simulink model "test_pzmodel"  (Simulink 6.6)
settings: Solver=ode45  StartTime=0.0  StopTime=10.0  RelTol=1e-3
libraries: sltpda x11

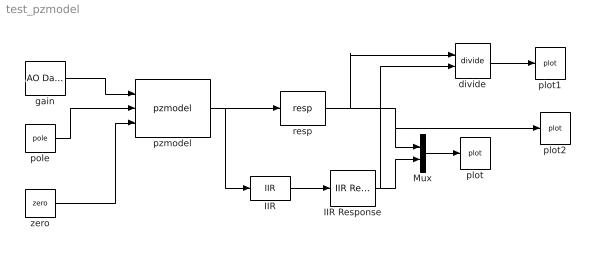
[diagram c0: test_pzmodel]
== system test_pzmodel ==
  IIR : sltpda/Pole//zero Modelling/IIR  SystemSampleTime=-1  fs=10000
  IIR Response : sltpda/Signal Processing blocks/Digital filtering/IIR Response  SystemSampleTime=-1  f1=0.1  f2=10000  nf=10000
  Mux : Mux  Inputs=2
  divide : sltpda/math blocks/divide  Tag=mrdivide  SystemSampleTime=-1
  gain : sltpda/AO class/AO Data  Tag=ao  SystemSampleTime=-1  vals=5
  plot : sltpda/AO class/plot  Tag=plot  Description=Plot an analysis object.  SystemSampleTime=-1  xscale=linear  yscale=linear
  plot1 : sltpda/AO class/plot  Tag=plot  Description=Plot an analysis object.  SystemSampleTime=-1  xscale=linear  yscale=linear
  plot2 : sltpda/AO class/plot  Tag=plot  Description=Plot an analysis object.  SystemSampleTime=-1  xscale=linear  yscale=linear
  pole : sltpda/Pole//zero Modelling/pole  Tag=pole  SystemSampleTime=-1  polef=1  poleQ=10
  pzmodel : sltpda/Pole//zero Modelling/pzmodel  SystemSampleTime=-1
  resp : sltpda/Pole//zero Modelling/resp  SystemSampleTime=-1  scale=linear
  zero : sltpda/Pole//zero Modelling/zero  Tag=zero  SystemSampleTime=-1  zerof=40  zeroQ=15
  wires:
  pole/1 -> pzmodel/2
  zero/1 -> pzmodel/3
  gain/1 -> pzmodel/1
  pzmodel/1 -> resp/1, IIR/1
  resp/1 -> divide/1, Mux/1, plot2/1
  IIR/1 -> IIR Response/1
  IIR Response/1 -> Mux/2, divide/2
  Mux/1 -> plot/1
  divide/1 -> plot1/1
